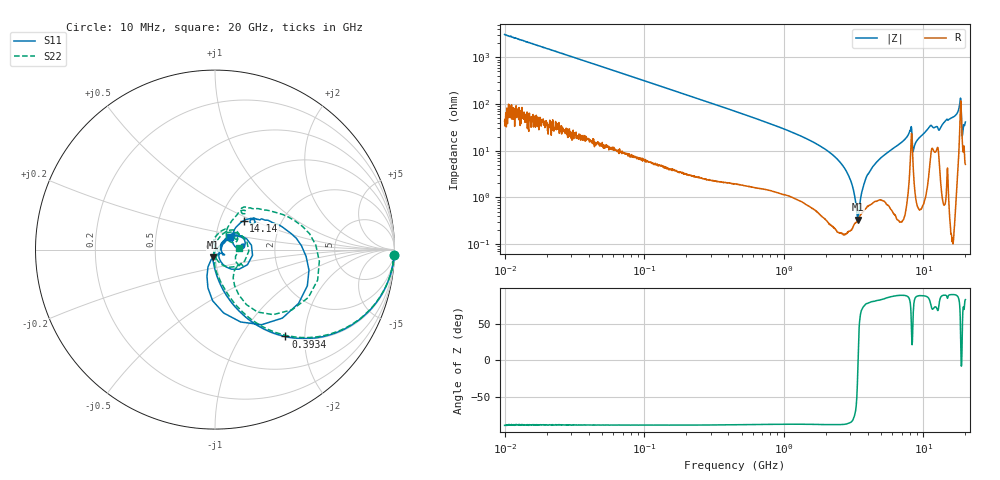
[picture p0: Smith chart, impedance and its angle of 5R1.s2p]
!Keysight Technologies,P5008B,MY61100088,A.16.20.02
!Date: Monday, November 06, 2023 16:03:14
!Correction: S11(C  2-Port  )
!S21(C  2-Port  )
!S12(C  2-Port  )
!S22(C  2-Port  )
!S2P File: Measurements: S11, S21, S12, S22:Log Frequency Sweep
# Hz S  dB  R 50
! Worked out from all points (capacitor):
!   1601 points, 10 MHz to 20 GHz, reference 50 ohm
!   read as one part in series: C = 5.14 pF near 10.39 MHz
!   lowest |Z| = 336 mohm at 3.4 GHz (marker M1)
!   series resonance near 3.404 GHz, so ESL is about 420 pH
!   S11 on the Smith chart (normalised r, x): 10 MHz: 2, -61; 393.4 MHz: 1.01, -1.60; 14.14 GHz: 1.30, +0.44; 20 GHz: 1.17, +0.16
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1e7  -0.01 -1.9  -29.82 87.3  -29.82 87.4  -0.01 -1.9
3.555162e7  -0.08 -6.5  -19.03 82.2  -19.03 82.2  -0.08 -6.5
1.263918e8  -0.69 -21.8  -8.68 67.1  -8.68 67.1  -0.70 -21.8
3.93378e8  -4.12 -51.0  -2.28 37.7  -2.29 37.7  -4.21 -50.7
4.472136e8  -4.82 -54.5  -1.88 34.1  -1.88 34.1  -4.95 -54.2
1.589917e9  -14.78 -82.5  -0.23 7.8  -0.23 7.8  -15.52 -81.4
3.399988e9  -27.07 -105.6  -0.09 -2.8  -0.09 -2.8  -25.01 -87.3
5.238699e9  -43.18 -72.1  -0.06 -9.4  -0.06 -9.5  -35.93 -13.7
5.652411e9  -44.23 -17.6  -0.05 -10.8  -0.05 -10.8  -38.18 36.5
7.410252e9  -24.17 45.8  -0.06 -17.5  -0.07 -17.5  -24.33 92.6
8.03353e9  -17.67 38.0  -0.46 -23.0  -0.47 -23.0  -18.62 54.2
8.305168e9  -15.26 -39.3  -1.40 -13.0  -1.40 -12.9  -16.32 -38.1
8.792373e9  -30.95 -36.4  -0.08 -17.8  -0.08 -17.8  -37.98 -121.6
9.046592e9  -31.78 -3.4  -0.04 -19.4  -0.04 -19.4  -42.03 133.6
9.761022e9  -26.87 29.5  -0.03 -22.9  -0.03 -22.9  -28.90 81.7
1.099193e10  -17.29 33.7  -0.35 -29.7  -0.35 -29.6  -17.66 54.4
1.304209e10  -19.51 23.5  -0.44 -27.5  -0.44 -27.5  -20.73 44.3
1.413906e10  -12.84 45.3  -0.22 -35.3  -0.22 -35.3  -12.95 57.8
1.726126e10  -9.62 29.8  -0.74 -52.8  -0.75 -52.8  -9.45 42.2
1.818725e10  -5.87 -4.3  -3.47 -67.2  -3.47 -67.3  -5.44 9.5
1.90721e10  -16.17 -106.7  -1.40 -31.1  -1.40 -31.0  -12.82 -61.5
2e10  -19.45 39.4  -0.58 -44.5  -0.58 -44.5  -17.41 3.2
